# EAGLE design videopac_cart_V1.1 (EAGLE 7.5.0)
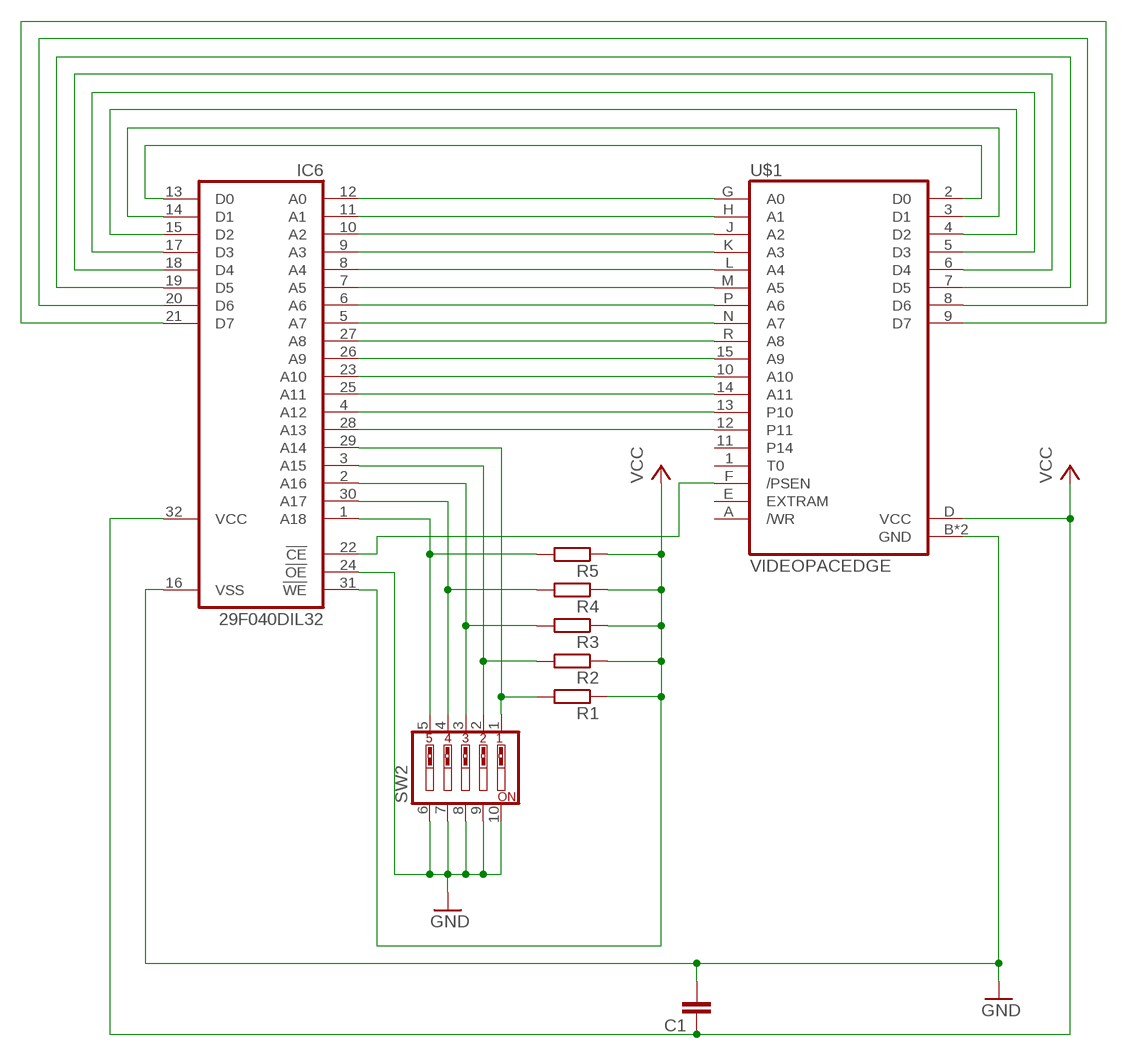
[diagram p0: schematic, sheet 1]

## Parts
C1  C-EU025-030X050  [C025-030X050]
IC6  29F040DIL32  [DIL32]
R1  R-EU_0207/10  [0207/10]
R2  R-EU_0207/10  [0207/10]
R3  R-EU_0207/10  [0207/10]
R4  R-EU_0207/10  [0207/10]
R5  R-EU_0207/10  [0207/10]
SW2  SW_DIP-5  [EDG-05]
U$1  VIDEOPACEDGE  [VIDEOPAC]

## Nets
GND [power]: C1.2 IC6.16(VSS) IC6.24(!OE) SW2.6 SW2.7 SW2.8 SW2.9 SW2.10 U$1.B(GND) U$1.C(GND)
N$1: IC6.12(A0) U$1.G(A0)
N$2: IC6.11(A1) U$1.H(A1)
N$3: IC6.10(A2) U$1.J(A2)
N$4: IC6.9(A3) U$1.K(A3)
N$5: IC6.8(A4) U$1.L(A4)
N$6: IC6.7(A5) U$1.M(A5)
N$7: IC6.6(A6) U$1.P(A6)
N$8: IC6.5(A7) U$1.N(A7)
N$9: IC6.27(A8) U$1.R(A8)
N$10: IC6.26(A9) U$1.15(A9)
N$11: IC6.23(A10) U$1.10(A10)
N$12: IC6.25(A11) U$1.14(A11)
N$13: IC6.4(A12) U$1.13(P10)
N$14: IC6.28(A13) U$1.12(P11)
N$15: IC6.29(A14) R1.2 SW2.1
N$16: IC6.3(A15) R2.2 SW2.2
N$17: IC6.2(A16) R3.2 SW2.3
N$18: IC6.30(A17) R4.2 SW2.4
N$19: IC6.1(A18) R5.2 SW2.5
N$20: IC6.22(!CE) U$1.F(/PSEN)
N$21: IC6.13(D0) U$1.2(D0)
N$22: IC6.14(D1) U$1.3(D1)
N$23: IC6.15(D2) U$1.4(D2)
N$24: IC6.17(D3) U$1.5(D3)
N$25: IC6.18(D4) U$1.6(D4)
N$26: IC6.19(D5) U$1.7(D5)
N$27: IC6.20(D6) U$1.8(D6)
N$28: IC6.21(D7) U$1.9(D7)
VCC [power]: C1.1 IC6.31(!WE) IC6.32(VCC) R1.1 R2.1 R3.1 R4.1 R5.1 U$1.D(VCC)
Unconnected: U$1.1(T0) U$1.11(P14) U$1.A(/WR) U$1.E(EXTRAM)

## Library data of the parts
C1 = rcl:C-EU: CAPACITOR, European symbol
IC6 = Mio:29F040
R1-R5 = rcl:R-EU_: RESISTOR, European symbol
SW2 = special:SW_DIP-5: DIP SWITCH
U$1 = BUSES:VIDEOPAC

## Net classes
0 default: width 0.406 mm
1 power: width 0.61 mm

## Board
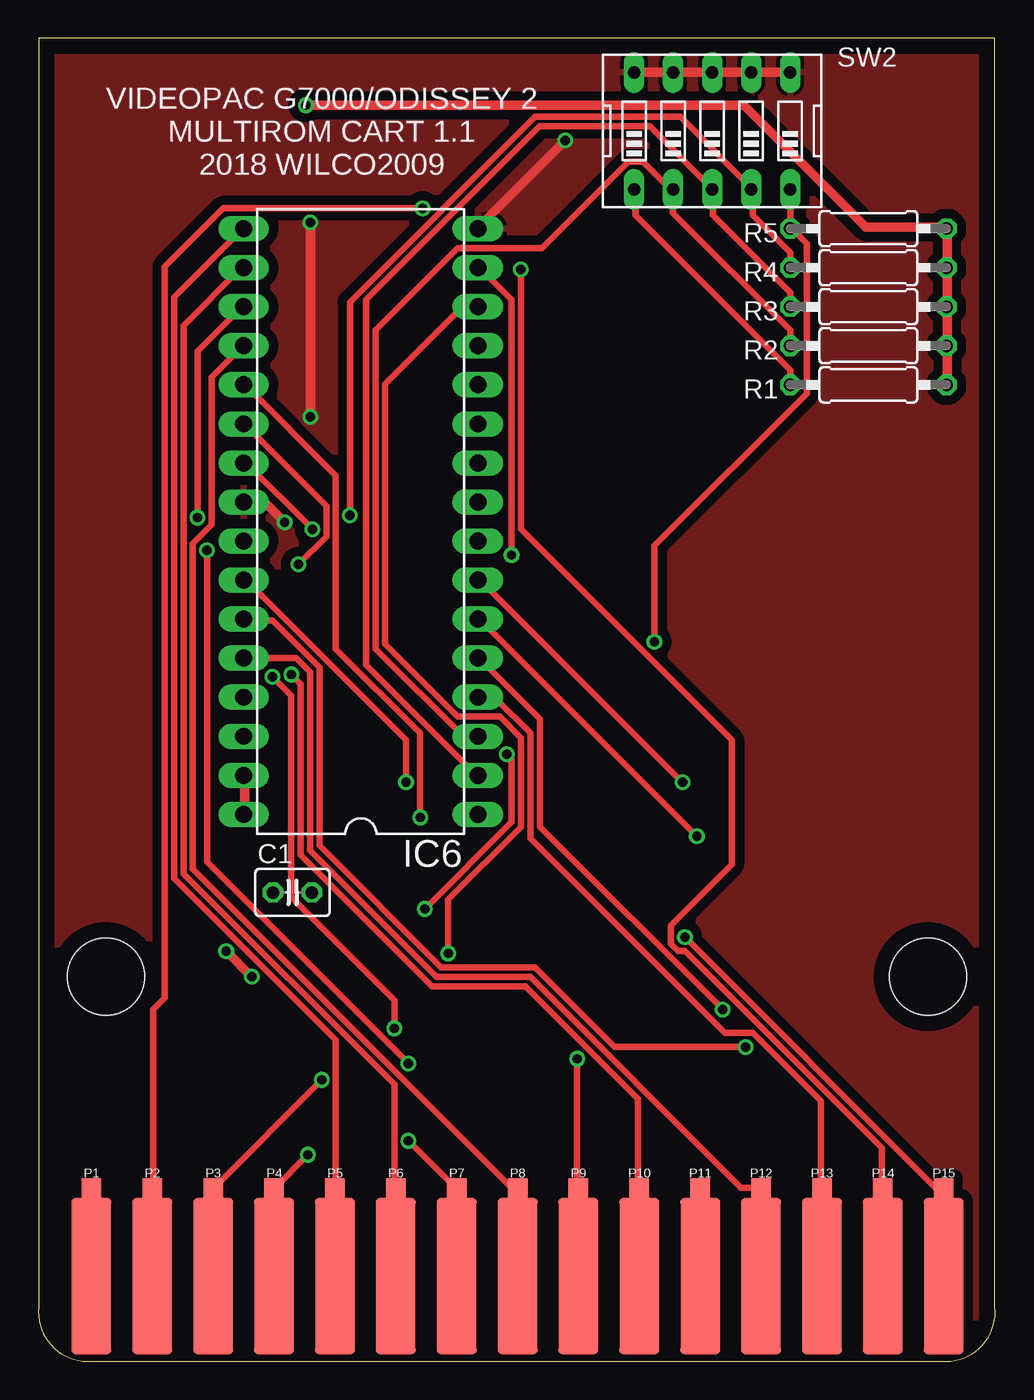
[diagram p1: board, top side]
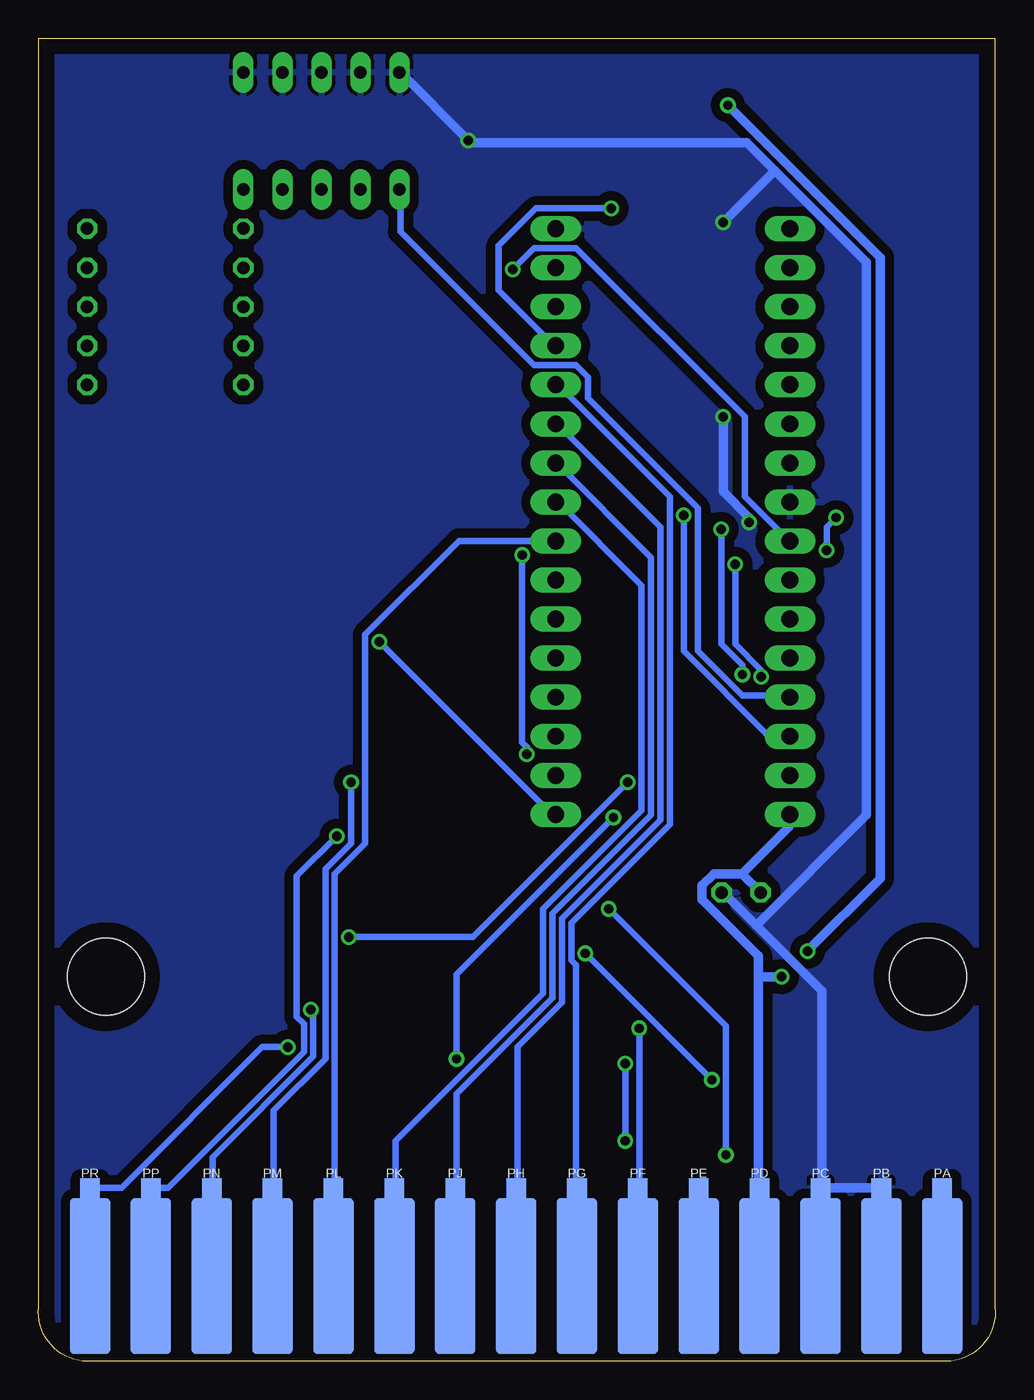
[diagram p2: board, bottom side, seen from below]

Size 62.24 x 86.03 mm. Coordinates in mm from the lower left corner, seen from the top.
Outline: 0.02,86.03 0.02,3.5 arc90 2.88,0 59.36,0 arc90 62.23,3.5 62.23,86.03 0.02,86.03
Copper layers (1*16): Top 0.035mm / dielectric 1.5mm / Bottom 0.035mm
Design rules "default *": minimum track width 16mil, minimum drill 24mil, track to track 8mil, track to pad 8mil, pad to pad 8mil, via to via 8mil, smd to smd 8mil, copper to edge 40mil, drill to drill 8mil, minimum pad ring 10mil, minimum via ring 8mil, stop-mask expansion 4mil, vias tented up to drill 0mil, thermal gap 10mil
Holes 5 mm at 4.38,25 57.86,25

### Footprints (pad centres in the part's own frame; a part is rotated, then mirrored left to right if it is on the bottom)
C025-030X050 = drill 0.813 octagon: 1 -1.27,0; 2 1.27,0
DIL32 = drill 1.1 long: 1 -21.59,-8.89; 2 -19.05,-8.89; 3 -16.51,-8.89; 4 -13.97,-8.89; 5 -11.43,-8.89; 6 -8.89,-8.89; 7 -6.35,-8.89; 8 -3.81,-8.89; 9 -1.27,-8.89; 10 1.27,-8.89; 11 3.81,-8.89; 12 6.35,-8.89; 13 8.89,-8.89; 14 11.43,-8.89; 15 13.97,-8.89; 16 16.51,-8.89; 17 16.51,6.35; 18 13.97,6.35; 19 11.43,6.35; 20 8.89,6.35; 21 6.35,6.35; 22 3.81,6.35; 23 1.27,6.35; 24 -1.27,6.35; 25 -3.81,6.35; 26 -6.35,6.35; 27 -8.89,6.35; 28 -11.43,6.35; 29 -13.97,6.35; 30 -16.51,6.35; 31 -19.05,6.35; 32 -21.59,6.35
0207/10 = drill 0.813 octagon: 1 -5.08,0; 2 5.08,0
EDG-05 = drill 0.813 long: 1 -5.08,-3.81; 2 -2.54,-3.81; 3 0,-3.81; 4 2.54,-3.81; 5 5.08,-3.81; 6 5.08,3.81; 7 2.54,3.81; 8 0,3.81; 9 -2.54,3.81; 10 -5.08,3.81
VIDEOPAC = smd 1.27 x 1.27: 1 -27.683,6.167; 2 -23.723,6.167; 3 -19.763,6.167; 4 -15.803,6.167; 5 -11.843,6.167; 6 -7.883,6.167; 7 -3.923,6.167; 8 0.037,6.167; 9 3.997,6.167; 10 7.957,6.167; 11 11.917,6.167; 12 15.877,6.167; 13 19.837,6.167; 14 23.797,6.167; 15 27.757,6.167 | smd 1.27 x 1.27 bottom: A -27.683,6.167; B -23.723,6.167; C -19.763,6.167; D -15.803,6.167; E -11.843,6.167; F -7.883,6.167; G -3.923,6.167; H 0.037,6.167; J 3.997,6.167; K 7.957,6.167; L 11.917,6.167; M 15.877,6.167; N 19.837,6.167; P 23.797,6.167; R 27.757,6.167 | smd 2.6 x 10.16: P$1 -27.683,0.452; P$2 -23.723,0.452; P$3 -19.763,0.452; P$4 -15.803,0.452; P$5 -11.843,0.452; P$6 -7.883,0.452; P$7 -3.923,0.452; P$8 0.037,0.452; P$9 3.997,0.452; P$10 7.957,0.452; P$11 11.917,0.452; P$12 15.877,0.452; P$13 19.837,0.452; P$14 23.797,0.452; P$15 27.757,0.452 | smd 2.6 x 10.16 bottom: P$A -27.683,0.452; P$B -23.723,0.452; P$C -19.763,0.452; P$D -15.803,0.452; P$E -11.843,0.452; P$F -7.883,0.452; P$H -3.923,0.452; P$J 0.037,0.452; P$K 3.997,0.452; P$L 7.957,0.452; P$M 11.917,0.452; P$N 15.877,0.452; P$P 19.837,0.452; P$R 23.797,0.452; P$S 27.757,0.452

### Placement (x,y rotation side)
C1  16.53,30.48 0 top
IC6  19.7,57.15 90 top
R1  53.99,63.5 180 top
R2  53.99,66.04 180 top
R3  53.99,68.58 180 top
R4  53.99,71.12 180 top
R5  53.99,73.66 180 top
SW2  43.83,80.01 0 top
U$1  31.13,5.08 0 top

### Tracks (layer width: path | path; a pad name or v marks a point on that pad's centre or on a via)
GND  (via drill 0.61)
  Top 0.61: SW2.10 SW2.9 SW2.8 SW2.7 SW2.6 | v34.28,79.4 28.64,73.76 IC6.16 | v16.02,54.56 14.65,55.93 13.43,55.93 IC6.24 | v17.69,74.07 v17.69,61.42
  Bottom 0.61: U$1.B 7.46,11.28 11.27,11.28 U$1.C 11.27,11.58 11.27,24.08 15.53,28.35 | 15.53,28.35 17.67,30.48 C1.2 | SW2.10 38.7,83.82 v34.28,79.4 34.13,79.25 16.14,79.25 14.33,77.43 | 15.53,28.35 8.37,35.51 8.37,71.48 14.33,77.43 | v16.02,54.56 16.02,54.86 17.69,56.54 v17.69,61.42 | 14.33,77.43 v17.69,74.07
  pour Bottom (isolate 0.61): 0.02,86.36 62.25,86.36 62.25,0 0.02,0
  pour Top (isolate 0.61): 0.02,86.36 62.25,86.36 62.25,0 0.02,0
N$1
  Bottom 0.406: U$1.G 27.27,11.28 27.27,25.76 27.57,26.06 27.57,28.5 21.17,34.9 21.17,56.24 28.49,63.55 IC6.12
N$2
  Bottom 0.406: U$1.H 31.08,11.28 31.08,20.42 28.18,23.32 28.18,28.8 21.78,35.2 21.78,54.25 28.49,60.96 IC6.11
N$3
  Bottom 0.406: U$1.J 35.04,11.28 35.04,17.37 28.79,23.62 28.79,29.11 22.39,35.51 22.39,52.27 28.49,58.37 IC6.10
N$4
  Bottom 0.406: U$1.K 39,11.28 39,14.33 29.4,23.93 29.4,29.41 23,35.81 23,50.44 28.49,55.93 IC6.9
N$5
  Bottom 0.406: IC6.8 34.89,53.34 40.99,47.24 40.99,33.68 42.97,31.7 42.97,11.28 U$1.L
N$6  (via drill 0.61)
  Top 0.406: v41.9,37.64 28.64,50.9 IC6.7
  Bottom 0.406: v41.9,37.64 41.9,33.68 43.58,32 43.58,19.66 46.93,16.31 46.93,11.28 U$1.M
N$7  (via drill 0.61)
  Top 0.406: v42.84,34.14 28.67,48.31 IC6.6
  Bottom 0.406: v42.84,34.14 45.43,31.55 45.43,22.4 44.97,21.95 44.97,20.12 53.81,11.28 54.88,11.28 U$1.P
N$8  (via drill 0.61)
  Top 0.406: v44.52,22.86 32.63,34.75 32.63,41.76 28.67,45.72 IC6.5
  Bottom 0.406: v44.52,22.86 44.36,22.71 44.36,19.81 50.92,13.26 50.92,11.28 U$1.N
N$9  (via drill 0.61)
  Top 0.406: v46.01,20.42 37.48,20.42 32.3,25.6 26.2,25.6 18.28,33.53 18.28,45.11 15.23,48.16 13.4,48.16 IC6.27
  Bottom 0.406: v46.01,20.42 47.69,20.42 56.84,11.28 58.82,11.28 U$1.R
N$10  (via drill 0.61)
  Top 0.406: v42.05,27.58 58.36,11.28 58.82,11.28 U$1.15 | v23.92,37.64 23.92,40.39 13.4,50.9 IC6.26
  Bottom 0.406: v42.05,27.58 33.98,27.58 v23.92,37.64
N$11  (via drill 0.61)
  Top 0.406: v16.45,44.65 17.06,44.04 17.06,32.92 25.59,24.38 31.69,24.38 39,17.07 39,11.28 U$1.10 | v17.82,54.1 13.4,58.52 IC6.23
  Bottom 0.406: v16.45,44.65 16.45,45.26 17.82,46.63 v17.82,54.1
N$12  (via drill 0.61)
  Top 0.406: v31.38,71.02 31.38,54.1 45.1,40.39 45.1,32.31 41.14,28.35 41.14,27.13 41.6,26.67 42.05,26.67 54.85,13.87 54.85,11.28 U$1.14
  Bottom 0.406: v31.38,71.02 30.01,72.39 27.27,72.39 16.3,61.42 16.3,56.24 13.4,53.34 IC6.25
N$13
  Top 0.406: U$1.13 50.89,11.28 50.89,16.92 46.47,21.34 44.64,21.34 31.99,33.98 31.99,40.84 29.71,43.13 28.64,43.13 IC6.4
N$14
  Top 0.406: IC6.28 16.75,45.72 17.67,44.81 17.67,33.22 25.9,24.99 31.99,24.99 45.71,11.28 46.93,11.28 U$1.12
N$15
  Top 0.406: R1.2 48.91,64.47 38.85,74.52 38.85,76.2 SW2.1
  Bottom 0.406: IC6.29 13.4,43.28 16.45,43.28 19.34,46.18 19.34,55.47 26.51,62.64 26.51,64.01 27.27,64.77 30.01,64.77 38.7,73.46 38.7,76.2 SW2.1
N$16
  Top 0.406: R2.2 48.91,67.06 41.29,74.68 SW2.2 41.14,76.2 39.31,78.03 38.39,78.03 32.76,72.39 27.27,72.39 21.94,67.06 21.94,46.33 27.57,40.69 28.49,40.69 IC6.3
N$17
  Top 0.406: R3.2 48.91,69.49 43.88,74.52 43.88,76.2 SW2.3 43.73,76.35 39.77,80.31 32.6,80.31 21.33,69.04 21.33,45.26 28.49,38.1 IC6.2
N$18  (via drill 0.61)
  Top 0.406: R4.2 48.91,72.08 46.47,74.52 46.47,76.2 SW2.4 46.32,76.35 41.75,80.92 32.3,80.92 20.26,68.89 v20.26,55.02
  Bottom 0.406: v20.26,55.02 20.26,46.18 14.77,40.69 13.4,40.69 IC6.30
N$19  (via drill 0.61)
  Top 0.406: SW2.5 R5.2 49.06,73.61 49.98,72.69 49.98,62.94 40.07,53.03 v40.07,46.79
  Bottom 0.406: v40.07,46.79 28.95,35.66 28.64,35.66 IC6.1
N$20  (via drill 0.61)
  Top 0.406: v23.15,21.64 23.15,23.47 16.45,30.18 16.45,43.28 v15.23,44.5 | v16.91,51.82 18.74,53.65 18.74,55.63 13.4,60.96 IC6.22
  Bottom 0.406: v23.15,21.64 23.15,11.28 U$1.F | v15.23,44.5 15.23,44.96 16.91,46.63 v16.91,51.82
N$21  (via drill 0.61)
  Top 0.406: v24.98,74.98 12.03,74.98 8.22,71.17 8.22,23.62 7.46,22.86 7.46,11.28 U$1.2
  Bottom 0.406: v24.98,74.98 29.86,74.98 32.3,72.54 32.3,69.65 28.64,65.99 IC6.13
N$22  (via drill 0.61)
  Top 0.406: v18.43,18.29 11.42,11.28 U$1.3 | v26.66,26.52 26.66,30.02 31.38,34.75 31.38,40.54 30.01,41.91 27.27,41.91 22.55,46.63 22.55,63.55 27.57,68.58 IC6.14
  Bottom 0.406: v26.66,26.52 v18.43,18.29
N$23  (via drill 0.61)
  Top 0.406: v17.52,13.41 15.38,11.28 U$1.4 | v25.14,29.41 30.77,35.05 30.77,39.17 v30.47,39.47 | v30.77,52.43 30.77,69.04 28.64,71.17 IC6.15
  Bottom 0.406: v17.52,13.41 17.52,21.79 v25.14,29.41 | v30.47,39.47 30.47,39.93 30.77,40.23 v30.77,52.43
N$24
  Top 0.406: U$1.5 19.34,11.28 19.34,20.88 8.83,31.39 8.83,69.19 13.25,73.61 IC6.17
N$25
  Top 0.406: U$1.6 23.15,11.28 23.15,17.98 9.44,31.7 9.44,67.36 13.25,71.17 IC6.18
N$26  (via drill 0.61)
  Top 0.406: v24.07,14.33 27.12,11.28 U$1.7 | v24.07,19.36 10.96,32.46 v10.96,52.73 | v10.35,54.86 10.35,65.68 13.25,68.58 IC6.19
  Bottom 0.406: v24.07,19.36 v24.07,14.33 | v10.96,52.73 10.96,54.25 v10.35,54.86
N$27
  Top 0.406: U$1.8 31.08,11.28 30.77,11.28 10.05,32 10.05,53.19 11.27,54.41 11.27,64.01 13.25,65.99 IC6.20
N$28  (via drill 0.61)
  Top 0.406: v35.04,19.66 35.04,11.28 U$1.9 | v24.83,35.36 24.83,40.84 19.34,46.33 19.34,57.61 13.4,63.55 IC6.21
  Bottom 0.406: v35.04,19.66 35.04,25.15 v24.83,35.36
VCC  (via drill 0.61)
  Top 0.61: R1.1 59.12,63.55 59.12,65.99 R2.1 59.12,66.29 59.12,68.58 R3.1 59.12,68.73 59.12,71.02 R4.1 59.12,71.32 59.12,73.61 R5.1 58.84,73.76 53.81,73.76 45.89,81.69 v17.39,81.69 | IC6.32 13.4,35.66 13.4,38.1 IC6.31 | v13.88,24.99 v12.21,26.67
  Bottom 0.61: 15.41,24.99 15.41,26.36 19.07,30.02 19.07,30.94 18.3,31.7 16.47,31.7 | 15.41,24.99 15.41,11.28 U$1.D | C1.1 16.47,31.7 | 16.47,31.7 13.43,34.75 13.43,35.51 IC6.32 | v17.39,81.69 7.48,71.78 7.48,31.39 v12.21,26.67 | 15.41,24.99 v13.88,24.99

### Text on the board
tPlace: VIDEOPAC G7000/ODISSEY 2 / MULTIROM CART 1.1 / 2018 WILCO2009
